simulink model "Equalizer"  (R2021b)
settings: Solver=ode1  StartTime=0.0  StopTime=10.0  FixedStep=0.1  RelTol=1e-3
undefined symbols (not defined in the file): dfilt, magnitude
libraries: dsparch4 x3, dspspect3 x1, dspmathops x1

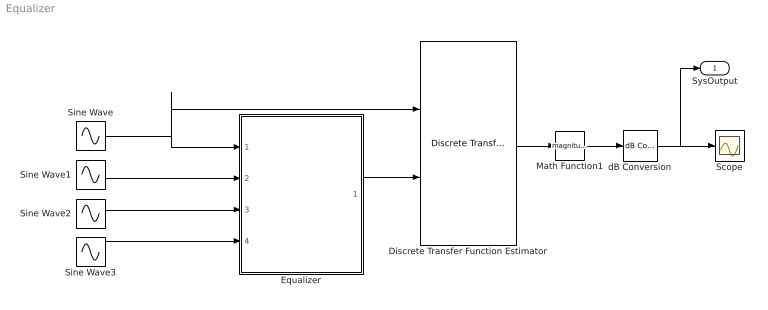
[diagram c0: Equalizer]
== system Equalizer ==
  Discrete Transfer Function Estimator : dspspect3/Discrete Transfer Function Estimator  WindowLength=1024  Overlap=0  AveragingMethod=Running  ForgettingFactorPort=off  ForgettingFactor=0.9  SpectralAverages=100  FFTLengthSource=Property  FFTLength=6  Window=Hann  SidelobeAttenuation=60  FrequencyRange=One-sided  OutputCoherence=off  SimulateUsing=Interpreted execution
  Equalizer : Subsystem  TreatAsAtomicUnit=on
  Math Function1 : Math  Operator=magnitude^2  SignedPower=on
  Scope : Scope
  Sine Wave : Sin  Amplitude=[1 2; 3 4; 5 6; 7 8; 9 10]  Phase=[1 2; 3 4; 5 6; 7 8; 9 10]  SampleTime=0.1
  Sine Wave1 : Sin  Phase=[1 2 3 4 5]  SampleTime=0.1
  Sine Wave2 : Sin  Phase=[6 7 8 9 10]  SampleTime=0.1
  Sine Wave3 : Sin  Amplitude=[1 0.5 0.25 0.5 1]  Phase=[11 12 13 14 15]  SampleTime=0.1
  dB Conversion : dspmathops/dB Conversion  dBtype=dB  intype=Power  R=1  fuzz=on
  SysOutput : Outport
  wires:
  Sine Wave3/1 -> Equalizer/4(coeffs3)
  Sine Wave2/1 -> Equalizer/3(coeffs2)
  Sine Wave1/1 -> Equalizer/2(coeffs1)
  Sine Wave/1 -> Discrete Transfer Function Estimator/1, Equalizer/1(In)
  Equalizer/1(Out) -> Discrete Transfer Function Estimator/2
  Discrete Transfer Function Estimator/1 -> Math Function1/1
  Math Function1/1 -> dB Conversion/1
  dB Conversion/1 -> Scope/1, SysOutput/1

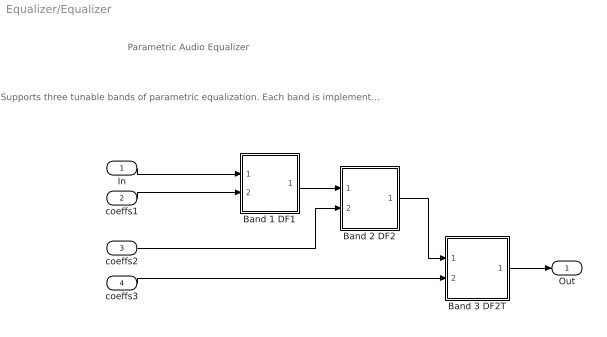
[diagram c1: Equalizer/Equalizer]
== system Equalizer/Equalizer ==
  note: Parametric Audio Equalizer
  note: Supports three tunable bands of parametric equalization. Each band is implemented using a different biquad filter structure Coefficients are slewed between changes..
  In : Inport
  coeffs1 : Inport  Port=2
  coeffs2 : Inport  Port=3
  coeffs3 : Inport  Port=4
  Band 1 DF1 : Subsystem  TreatAsAtomicUnit=on
  Band 2 DF2 : Subsystem  TreatAsAtomicUnit=on
  Band 3 DF2T : Subsystem  TreatAsAtomicUnit=on
  Out : Outport  VectorParamsAs1DForOutWhenUnconnected=off
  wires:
  In/1 -> Band 1 DF1/1(In)
  coeffs2/1 -> Band 2 DF2/2(coeffs)
  Band 1 DF1/1(Out) -> Band 2 DF2/1(In)
  Band 2 DF2/1(Out) -> Band 3 DF2T/1(In)
  Band 3 DF2T/1(Out) -> Out/1
  coeffs1/1 -> Band 1 DF1/2(coeffs)
  coeffs3/1 -> Band 3 DF2T/2(coeffs)

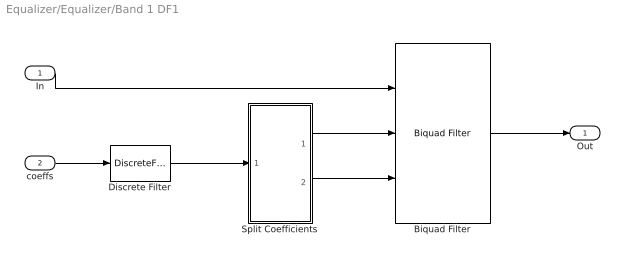
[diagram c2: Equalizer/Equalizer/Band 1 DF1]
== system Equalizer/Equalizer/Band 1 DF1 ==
  In : Inport
  coeffs : Inport  Port=2
  Biquad Filter : dsparch4/Biquad Filter  FilterSource=Input port(s)  CoeffSource=Specify via dialog  FilterObject=dfilt.df2tsos([1 0.3 0.4],[1 0.1 0.2])  IIRFiltStruct=Direct form I  BiQuadCoeffs=[1 0.3 0.4 1 0.1 0.2]  ScaleValues=1  IC=0  ICnum=0  ICden=0  a0Flag=Warning  optimizeScaleValues=on  ScaleValueMode=Assume all are unity and optimize  InputProcessing=Columns as channels (frame based)  roundingMode=Floor  overflowMode=off  scaleValueFracLength=14  denProdOutputFracLength=30  denAccumFracLength=30  secondMemoryFracLength=15
  Discrete Filter : DiscreteFilter  Numerator=[.25]  Denominator=[1 -.75]
  Split Coefficients : Subsystem
  Out : Outport  VectorParamsAs1DForOutWhenUnconnected=off
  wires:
  Biquad Filter/1 -> Out/1
  In/1 -> Biquad Filter/1
  Discrete Filter/1 -> Split Coefficients/1(In)
  coeffs/1 -> Discrete Filter/1
  Split Coefficients/2(Den) -> Biquad Filter/3
  Split Coefficients/1(Num) -> Biquad Filter/2

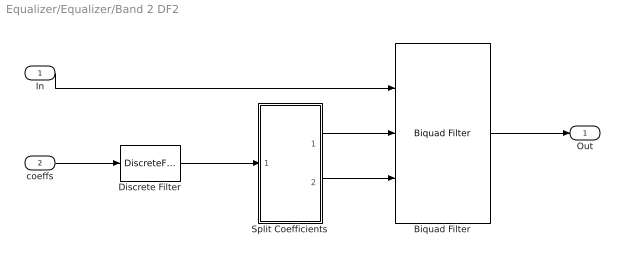
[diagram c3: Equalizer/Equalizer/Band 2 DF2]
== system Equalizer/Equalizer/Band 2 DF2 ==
  In : Inport
  coeffs : Inport  Port=2
  Biquad Filter : dsparch4/Biquad Filter  FilterSource=Input port(s)  CoeffSource=Specify via dialog  FilterObject=dfilt.df2tsos([1 0.3 0.4],[1 0.1 0.2])  IIRFiltStruct=Direct form I  BiQuadCoeffs=[1 0.3 0.4 1 0.1 0.2]  ScaleValues=1  IC=0  ICnum=0  ICden=0  a0Flag=Warning  optimizeScaleValues=on  ScaleValueMode=Assume all are unity and optimize  InputProcessing=Columns as channels (frame based)  roundingMode=Floor  overflowMode=off  scaleValueFracLength=14  denProdOutputFracLength=30  denAccumFracLength=30  secondMemoryFracLength=15
  Discrete Filter : DiscreteFilter  Numerator=[.25]  Denominator=[1 -.75]
  Split Coefficients : Subsystem
  Out : Outport  VectorParamsAs1DForOutWhenUnconnected=off
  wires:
  Biquad Filter/1 -> Out/1
  In/1 -> Biquad Filter/1
  Discrete Filter/1 -> Split Coefficients/1(In)
  Split Coefficients/2(Den) -> Biquad Filter/3
  Split Coefficients/1(Num) -> Biquad Filter/2
  coeffs/1 -> Discrete Filter/1

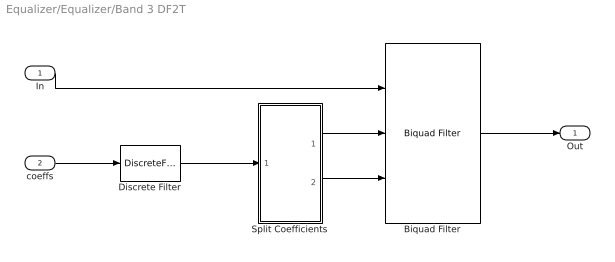
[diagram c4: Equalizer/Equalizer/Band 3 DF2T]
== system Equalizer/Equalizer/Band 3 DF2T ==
  In : Inport
  coeffs : Inport  Port=2
  Biquad Filter : dsparch4/Biquad Filter  FilterSource=Input port(s)  CoeffSource=Specify via dialog  FilterObject=dfilt.df2tsos([1 0.3 0.4],[1 0.1 0.2])  IIRFiltStruct=Direct form I  BiQuadCoeffs=[1 0.3 0.4 1 0.1 0.2]  ScaleValues=1  IC=0  ICnum=0  ICden=0  a0Flag=Warning  optimizeScaleValues=on  ScaleValueMode=Assume all are unity and optimize  InputProcessing=Columns as channels (frame based)  roundingMode=Floor  overflowMode=off  scaleValueFracLength=14  denProdOutputFracLength=30  denAccumFracLength=30  secondMemoryFracLength=15
  Discrete Filter : DiscreteFilter  Numerator=[.25]  Denominator=[1 -.75]
  Split Coefficients : Subsystem
  Out : Outport  VectorParamsAs1DForOutWhenUnconnected=off
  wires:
  Biquad Filter/1 -> Out/1
  In/1 -> Biquad Filter/1
  Discrete Filter/1 -> Split Coefficients/1(In)
  Split Coefficients/1(Num) -> Biquad Filter/2
  Split Coefficients/2(Den) -> Biquad Filter/3
  coeffs/1 -> Discrete Filter/1

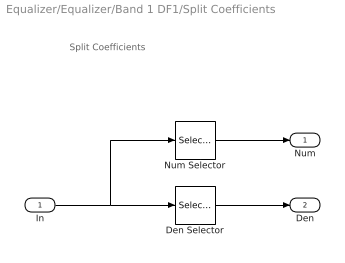
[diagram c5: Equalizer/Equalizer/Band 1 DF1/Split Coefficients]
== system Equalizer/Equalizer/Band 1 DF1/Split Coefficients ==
  note: Split Coefficients
  In : Inport
  Den Selector : Selector  InputPortWidth=5  IndexOptions=Index vector (dialog)  Indices=[4 5]  OutputSizes=1
  Num Selector : Selector  InputPortWidth=5  IndexOptions=Index vector (dialog)  Indices=[1 2 3]  OutputSizes=1
  Num : Outport  VectorParamsAs1DForOutWhenUnconnected=off
  Den : Outport  Port=2  VectorParamsAs1DForOutWhenUnconnected=off
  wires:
  In/1 -> Num Selector/1, Den Selector/1
  Num Selector/1 -> Num/1
  Den Selector/1 -> Den/1

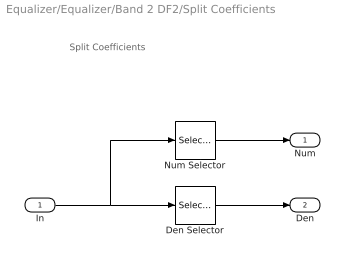
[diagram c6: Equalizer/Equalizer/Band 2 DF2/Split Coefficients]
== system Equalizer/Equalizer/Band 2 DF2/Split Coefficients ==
  note: Split Coefficients
  In : Inport
  Den Selector : Selector  InputPortWidth=5  IndexOptions=Index vector (dialog)  Indices=[4 5]  OutputSizes=1
  Num Selector : Selector  InputPortWidth=5  IndexOptions=Index vector (dialog)  Indices=[1 2 3]  OutputSizes=1
  Num : Outport  VectorParamsAs1DForOutWhenUnconnected=off
  Den : Outport  Port=2  VectorParamsAs1DForOutWhenUnconnected=off
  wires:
  In/1 -> Num Selector/1, Den Selector/1
  Num Selector/1 -> Num/1
  Den Selector/1 -> Den/1

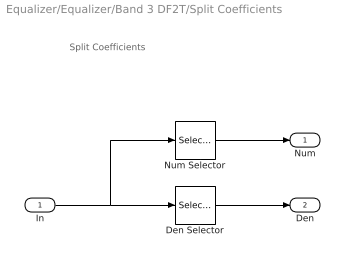
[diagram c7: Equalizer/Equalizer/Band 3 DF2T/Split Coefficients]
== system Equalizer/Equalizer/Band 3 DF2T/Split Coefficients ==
  note: Split Coefficients
  In : Inport
  Den Selector : Selector  InputPortWidth=5  IndexOptions=Index vector (dialog)  Indices=[4 5]  OutputSizes=1
  Num Selector : Selector  InputPortWidth=5  IndexOptions=Index vector (dialog)  Indices=[1 2 3]  OutputSizes=1
  Num : Outport  VectorParamsAs1DForOutWhenUnconnected=off
  Den : Outport  Port=2  VectorParamsAs1DForOutWhenUnconnected=off
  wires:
  In/1 -> Num Selector/1, Den Selector/1
  Num Selector/1 -> Num/1
  Den Selector/1 -> Den/1
